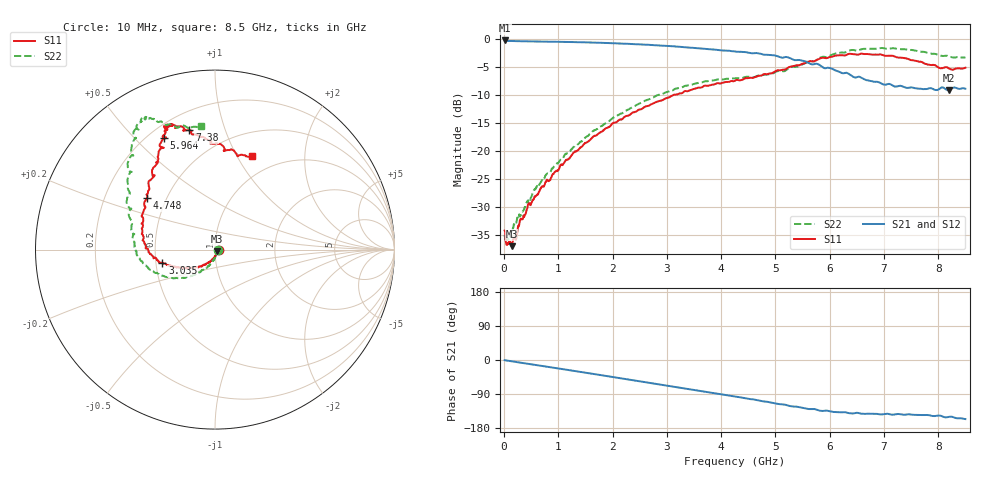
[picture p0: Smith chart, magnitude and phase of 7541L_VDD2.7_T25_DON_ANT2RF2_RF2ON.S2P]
!Agilent Technologies,E5071C,MY46417908,A.11.23
!Date: Wed Dec 09 17:17:37 2020
!Data & Calibration Information:
!Freq	S11:SOLT2(ON)	S21:SOLT2(ON)	S12:SOLT2(ON)	S22:SOLT2(ON)
!PortZ  Port1:50+j0  Port2:50+j0
!Above PortZ is port z conversion or system Z0 setting when saving the data.
!When reading, reference impedance value at option line is always used.
# Hz S dB R 50
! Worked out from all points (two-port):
!   1601 points, 10 MHz to 8.5 GHz, reference 50 ohm
!   highest |S21| = -0.20 dB at 10 MHz (marker M1); lowest = -9.1 dB at 8.198 GHz (marker M2)
!   |S21| within 3 dB of the highest: start of sweep to 5.094 GHz; 5.162 GHz to 5.225 GHz (62.97 MHz wide, 1.21 % of centre)
!   lowest |S11| = -36.9 dB at 137.3 MHz (marker M3), VSWR 1.03, Z = 51 - j1.07 ohm
!   |S11| at or under -10 dB: start of sweep to 3.108 GHz
!   |S22| runs from -36.0 to -1.5 dB; largest |S21 - S12| = 0.0038
!   S11 on the Smith chart (normalised r, x): 10 MHz: 1.04, -0.00; 3.035 GHz: 0.54, -0.09; 4.748 GHz: 0.39, +0.29; 5.964 GHz: 0.26, +0.61; 7.38 GHz: 0.31, +0.76; 8.5 GHz: 0.76, +1.15
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1e7  -34.15 -2.7  -0.20 -0.5  -0.20 -0.5  -35.27 -13.4
7.3675e7  -36.39 -31.1  -0.28 -1.9  -0.28 -1.9  -35.62 -33.4
1.3735e8  -36.95 -47.7  -0.29 -3.4  -0.29 -3.4  -34.20 -44.5
1.904125e8  -35.37 -57.6  -0.30 -4.6  -0.31 -4.5  -32.99 -53.8
4.398062e8  -29.53 -81.5  -0.35 -10.1  -0.35 -10.1  -29.13 -82.2
6.785875e8  -26.60 -97.4  -0.39 -15.2  -0.39 -15.2  -25.43 -93.5
1.426769e9  -19.21 -127.0  -0.52 -31.8  -0.52 -31.8  -18.23 -118.9
2.015762e9  -14.91 -143.9  -0.69 -45.1  -0.70 -45.1  -13.96 -132.6
2.843538e9  -11.07 -162.0  -1.09 -64.2  -1.09 -64.2  -9.93 -152.2
3.034562e9  -10.39 -165.9  -1.18 -68.6  -1.19 -68.6  -9.31 -156.7
3.734988e9  -8.28 178.5  -1.73 -84.7  -1.73 -84.7  -7.48 -173.1
4.255e9  -7.38 160.6  -2.17 -96.7  -2.17 -96.6  -6.96 177.0
4.748481e9  -6.45 142.7  -2.63 -108.6  -2.62 -108.6  -6.35 165.4
5.257881e9  -4.94 128.1  -3.31 -121.2  -3.30 -121.2  -5.06 151.9
5.671769e9  -3.93 117.3  -4.47 -129.4  -4.43 -129.4  -3.90 137.3
5.963612e9  -3.29 114.5  -5.06 -134.0  -5.05 -133.9  -3.12 131.1
6.425256e9  -2.64 110.0  -6.64 -141.1  -6.67 -140.8  -1.89 123.1
7.088538e9  -2.93 108.2  -7.95 -142.6  -7.96 -142.8  -1.68 118.3
7.380381e9  -3.35 102.1  -8.56 -144.5  -8.56 -144.3  -1.76 116.1
7.884475e9  -4.60 90.6  -8.79 -147.6  -8.80 -147.6  -2.58 111.2
8.197544e9  -5.21 77.7  -9.09 -150.1  -9.13 -150.1  -3.04 103.4
8.5e9  -5.07 68.4  -8.81 -155.9  -8.87 -156.0  -3.21 96.6
